(* Logix 5000 AddOnInstructionDefinition export AMCI_MAH; software revision 20.05 *)

TYPE AMCI_Motion_Axis_Output_Data :
STRUCT
   Control_Word_0 : INT;
   Control_Word_1 : INT;
   Position_or_Distance : DINT;
   Programmed_Speed : DINT;
   Acceleration : INT;
   Deceleration : INT;
   Output_Word_8 : INT;
   Output_Word_9 : INT;
END_STRUCT
END_TYPE

TYPE AMCI_Motion_Axis_Input_Data :
STRUCT
   Moving_CW : BOOL;
   Moving_CCW : BOOL;
   In_Hold_State : BOOL;
   Stopped : BOOL;
   At_Home : BOOL;
   Accelerating : BOOL;
   Decelerating : BOOL;
   Move_Complete : BOOL;
   Status_Word_0_Bit_8 : BOOL;
   Status_Word_0_Bit_9 : BOOL;
   Position_Invalid : BOOL;
   Input_Error : BOOL;
   Command_Error : BOOL;
   Configuration_Error : BOOL;
   Module_OK : BOOL;
   Mode_Flag : BOOL;
   IN1_Active : BOOL;
   IN2_Active : BOOL;
   IN3_Active : BOOL;
   IN4_Active : BOOL;
   Status_Word_1_Bit_4 : BOOL;
   Status_Word_1_Bit_5 : BOOL;
   Connection_Was_Lost : BOOL;
   Driver_Fault : BOOL;
   Status_Word_1_Bit_8 : BOOL;
   Invalid_Jog_Change : BOOL;
   Status_Word_1_Bit_10 : BOOL;
   Heartbeat_Bit : BOOL;
   Status_Word_1_Bit_12 : BOOL;
   Status_Word_1_Bit_13 : BOOL;
   Stall_Detected : BOOL;
   Drive_Is_Enabled : BOOL;
   Motor_Position : DINT;
   Encoder_Position : DINT;
   Trapped_Encoder_Position : DINT;
   Input_Word_8 : INT;
   Input_Word_9 : INT;
END_STRUCT
END_TYPE

ADD_ON_INSTRUCTION AMCI_MAH   (* revision 1.0, vendor AMCI, ExecuteEnableInFalse *)
// AMCI Motion Axis Home
// Revision note:
// 11/28/22 Initial release of AOI
// Help:
// MOTION AXIS HOME:   Performs CW or CCW Home Moves to a Home Input.
// AXIS INPUT DATA:  Input data from AMCI motion device.   Uses the AMCI_Motion_Axis_Input_Data User Defined Data Type.
// AXIS OUTPUT DATA; Output data from the AOI to the AMCI motion device.   Uses the AMCI_Motion_Axis_Output_Data User Defined Data Type.
// DIRECTION: 0 = CW Home, 1 = CCW Home
// PROGRAMMED SPEED: Speed of move in units of steps / sec
// ACCELERATION: Acceleration Rate in units of steps / sec / ms
// DECELERATION:  Deceleration Rate in units of steps / sec / ms
// EN (Enable) Set when rung is true, Reset when rung is false
// DN (Done) Set when command is sent to the motion device.  Reset when the rung is false.
// ER (Error) Set when a command or input error failed to clear.  Reset when the rung is false.
// IP (In Process) Set when motion is occurring.   Reset when motion stops or the rung goes false.
// PC (Process Complete) Set when the At Home Status bit is set.   Reset the next time the rung with the AOI                                      goes from false to true.
VAR_IN_OUT
   Axis_Input_Data : AMCI_Motion_Axis_Input_Data; {required}
        [0].6   // set when decelerating
   Axis_Output_Data : AMCI_Motion_Axis_Output_Data; {required}
END_VAR
VAR_INPUT
   Direction_0_CW_1_CCW : BOOL; {required}   // 0=home CW 1=home CCW
   Programmed_Speed : DINT; {required}
   Acceleration : INT; {required}
   Deceleration : INT; {required}
END_VAR
VAR_OUTPUT
   EN : BOOL; {visible}   // set when rung with AOI is true
   DN : BOOL; {access Read Only, visible}   // set when move was succesfully initiated
   ER : BOOL; {visible}   // input, command, or configuration error
   IP : BOOL; {visible}   // set when motion occurring
   PC : BOOL; {visible}   // set when process complete
END_VAR
VAR
   command_data_block : INT[10];
        [0]   // Command Bits MSW
        [1]   // Command Bits LSW
        [2]   // Upper Target Position
        [3]   // Lower Target Position
        [4]   // Upper Programmed Speed
        [5]   // Lower Programmed Speed
   motion_occurring : BOOL; {access None}
   Internal_Enable : BOOL; {access None}   // set when driver ready to receive motion command
END_VAR

ROUTINE EnableInFalse   (* ladder *)
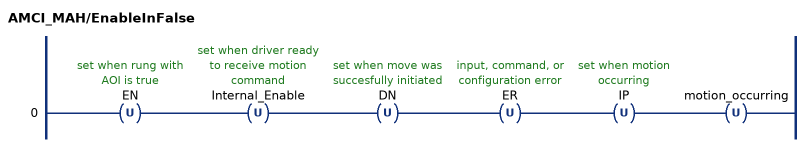
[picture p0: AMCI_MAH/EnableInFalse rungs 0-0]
   0: OTU(EN)OTU(Internal_Enable)OTU(DN)OTU(ER)OTU(IP)OTU(motion_occurring);
END_ROUTINE

ROUTINE Logic   (* ladder *)
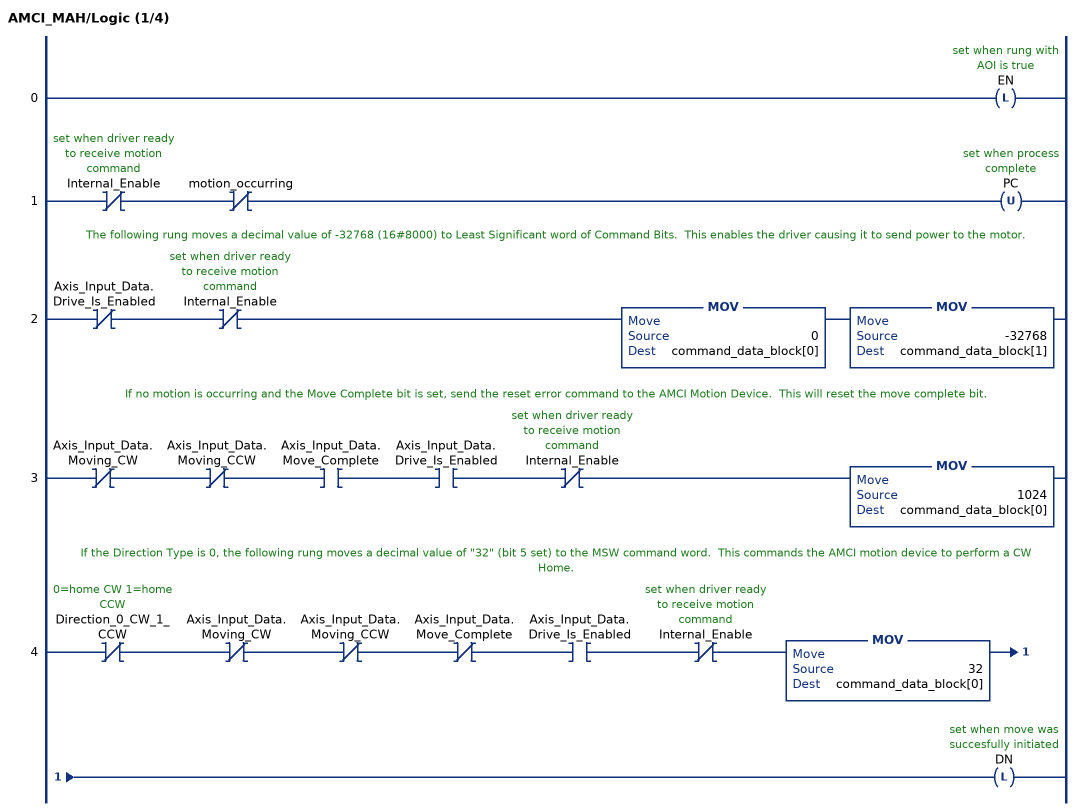
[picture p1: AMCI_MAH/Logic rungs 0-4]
   0: OTL(EN);
   1: XIO(Internal_Enable)XIO(motion_occurring)OTU(PC);
   // The following rung moves a decimal value of -32768 (16#8000) to Least Significant word of Command Bits.  This enables the driver causing it to send power to the motor.
   2: XIO(Axis_Input_Data.Drive_Is_Enabled)XIO(Internal_Enable)MOV(0,command_data_block[0])MOV(-32768,command_data_block[1]);
   // If no motion is occurring and the Move Complete bit is set, send the reset error command to the AMCI Motion Device.  This will reset the move complete bit.
   3: XIO(Axis_Input_Data.Moving_CW)XIO(Axis_Input_Data.Moving_CCW)XIC(Axis_Input_Data.Move_Complete)XIC(Axis_Input_Data.Drive_Is_Enabled)XIO(Internal_Enable)MOV(1024,command_data_block[0]);
   // If the Direction Type is 0, the following rung moves a decimal value of "32" (bit 5 set) to the MSW command word.  This commands the AMCI motion device to perform a CW Home.
   4: XIO(Direction_0_CW_1_CCW)XIO(Axis_Input_Data.Moving_CW)XIO(Axis_Input_Data.Moving_CCW)XIO(Axis_Input_Data.Move_Complete)XIC(Axis_Input_Data.Drive_Is_Enabled)XIO(Internal_Enable)MOV(32,command_data_block[0])OTL(DN);
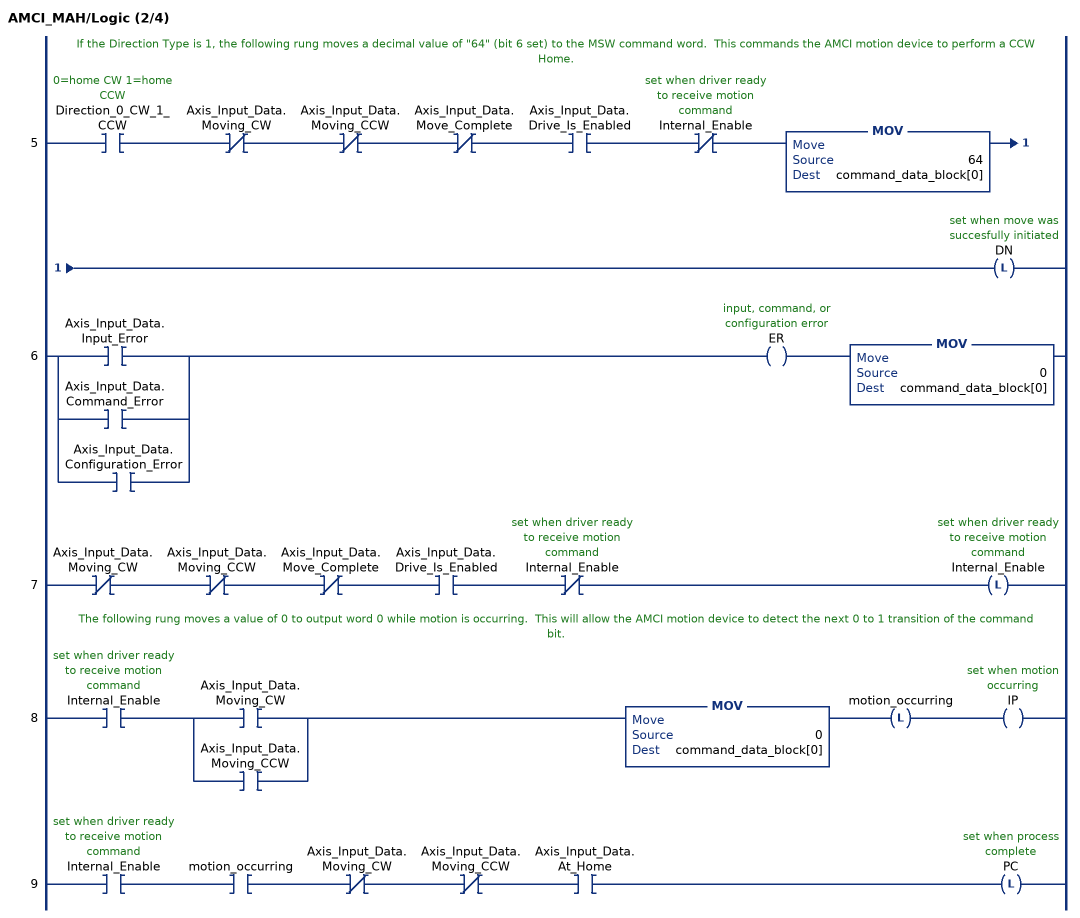
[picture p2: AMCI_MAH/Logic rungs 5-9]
   // If the Direction Type is 1, the following rung moves a decimal value of "64" (bit 6 set) to the MSW command word.  This commands the AMCI motion device to perform a CCW Home.
   5: XIC(Direction_0_CW_1_CCW)XIO(Axis_Input_Data.Moving_CW)XIO(Axis_Input_Data.Moving_CCW)XIO(Axis_Input_Data.Move_Complete)XIC(Axis_Input_Data.Drive_Is_Enabled)XIO(Internal_Enable)MOV(64,command_data_block[0])OTL(DN);
   6: [XIC(Axis_Input_Data.Input_Error) ,XIC(Axis_Input_Data.Command_Error) ,XIC(Axis_Input_Data.Configuration_Error) ]OTE(ER)MOV(0,command_data_block[0]);
   7: XIO(Axis_Input_Data.Moving_CW)XIO(Axis_Input_Data.Moving_CCW)XIO(Axis_Input_Data.Move_Complete)XIC(Axis_Input_Data.Drive_Is_Enabled)XIO(Internal_Enable)OTL(Internal_Enable);
   // The following rung moves a value of 0 to output word 0 while motion is occurring.  This will allow the AMCI motion device to detect the next 0 to 1 transition of the command bit.
   8: XIC(Internal_Enable)[XIC(Axis_Input_Data.Moving_CW) ,XIC(Axis_Input_Data.Moving_CCW) ]MOV(0,command_data_block[0])OTL(motion_occurring)OTE(IP);
   9: XIC(Internal_Enable)XIC(motion_occurring)XIO(Axis_Input_Data.Moving_CW)XIO(Axis_Input_Data.Moving_CCW)XIC(Axis_Input_Data.At_Home)OTL(PC);
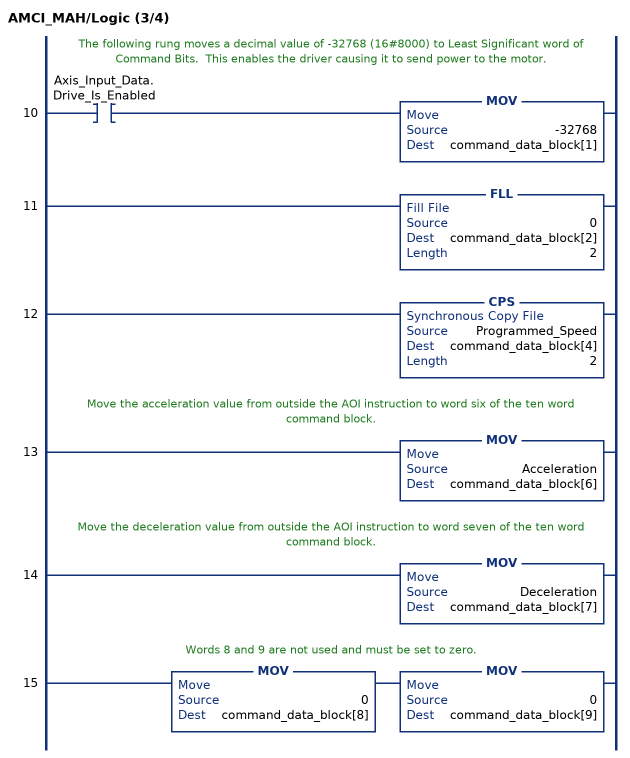
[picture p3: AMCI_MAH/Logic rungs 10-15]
   // The following rung moves a decimal value of -32768 (16#8000) to Least Significant word of Command Bits.  This enables the driver causing it to send power to the motor.
   10: XIC(Axis_Input_Data.Drive_Is_Enabled)MOV(-32768,command_data_block[1]);
   11: FLL(0,command_data_block[2],2);
   12: CPS(Programmed_Speed,command_data_block[4],2);
   // Move the acceleration value from outside the AOI instruction to word six of the ten word command block.
   13: MOV(Acceleration,command_data_block[6]);
   // Move the deceleration value from outside the AOI instruction to word seven of the ten word command block.
   14: MOV(Deceleration,command_data_block[7]);
   // Words 8 and 9 are not used and must be set to zero.
   15: MOV(0,command_data_block[8])MOV(0,command_data_block[9]);
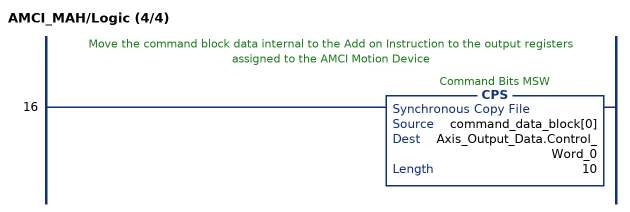
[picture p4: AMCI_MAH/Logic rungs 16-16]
   // Move the command block data internal to the Add on Instruction to the output registers assigned to the AMCI Motion Device
   16: CPS(command_data_block[0],Axis_Output_Data.Control_Word_0,10);
END_ROUTINE
END_ADD_ON_INSTRUCTION
